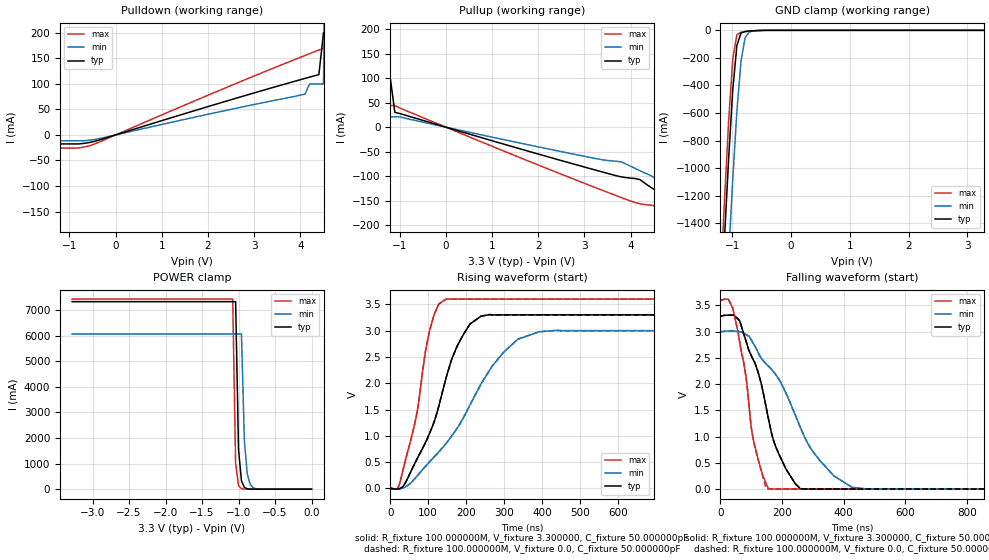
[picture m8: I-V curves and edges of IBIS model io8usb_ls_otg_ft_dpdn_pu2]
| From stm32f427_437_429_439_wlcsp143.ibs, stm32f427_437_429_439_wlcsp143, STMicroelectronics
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|   Model io8usb_ls_otg_ft_dpdn_pu2
[Model]  io8usb_ls_otg_ft_dpdn_pu2
Model_type I/O
Polarity   Non-Inverting
Enable   Active-Low
Vinl =   0.990000V
Vinh =   2.310000V
Vmeas =  1.650000V
Cref =   50.000000pF
Rref =   100.000000M
Vref =   0.0V
C_comp   8.255900pF   7.991100pF   8.650600pF
[Temperature Range]   25.000000   0.125000k   -40.000000
[Pullup Reference]   3.300000V   3.000000V   3.600000V
[Pulldown Reference]   0.0V   0.0V   0.0V
[POWER Clamp Reference]   3.300000V   3.000000V   3.600000V
[GND Clamp Reference]   0.0V   0.0V   0.0V
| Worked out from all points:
|   slope of the pulldown table from 0 to 0.495 V, typ, clamps not added: 35.6 ohm
|   slope of the pullup table from 0 to 0.495 V, typ, clamps not added: 36 ohm
|   GND clamp passes 1 mA (typ) near -0.52 V on its own axis
|   POWER clamp passes 1 mA (typ) near -0.81 V on its own axis
|   rising waveform, R_fixture 100.000000M, V_fixture 3.300000, C_fixture 50.000000pF: 20-80 % time 94.8ns typ, 161ns min, 53.8ns max; typ from 0 V to 3.3 V
|   rising waveform, R_fixture 100.000000M, V_fixture 0.0, C_fixture 50.000000pF: 20-80 % time 94.8ns typ, 162ns min, 53.7ns max; typ from 0 V to 3.3 V
|   falling waveform, R_fixture 100.000000M, V_fixture 3.300000, C_fixture 50.000000pF: 20-80 % time 97.5ns typ, 169ns min, 55.3ns max; typ from 3.3 V to 0 V
|   falling waveform, R_fixture 100.000000M, V_fixture 0.0, C_fixture 50.000000pF: 20-80 % time 97.5ns typ, 169ns min, 55.3ns max; typ from 3.3 V to 0 V
[Pulldown]
|Voltage   I(typ)   I(min)   I(max)
-3.3V     -181mA     -11.47mA   -25.86mA
-3.2V     -17.62mA   -11.47mA   -25.86mA
-600mV    -15.36mA   -10.76mA   -22.01mA
4.1V      110.7mA    80mA       155.6mA
4.2V      113.2mA    100mA      159.2mA
4.4V      118mA      100mA      166.2mA
4.5V      200mA      100mA      169.7mA
4.6V      200mA      1A         173.2mA
4.7V      200mA      1A         177mA
4.8V      1A         1A         200mA
5.4V      1A         1A         1A
6.6V      1A         1A         1A
[Pullup]
|Voltage   I(typ)   I(min)   I(max)
-3.3V     1A         1A         1A
-1.9V     1A         1A         1A
-1.8V     100mA      1A         1A
-1.7V     100mA      1A         100mA
-1.6V     100mA      1A         100mA
-1.5V     100mA      21mA       100mA
-1.3V     100mA      21mA       100mA
-1.2V     100mA      21mA       44mA
-1.1V     30mA       21mA       44mA
3.8V      -101.5mA   -71.06mA   -143.6mA
5V        -156.5mA   -125mA     -203mA
6.6V      -223mA     -162mA     -321mA
[GND_clamp]
|Voltage   I(typ)   I(min)   I(max)
-3.3V     -9.433A    -9.435A    -9.911A
-1.2V     -2.116A    -2.846A    -1.847A
-1.13V    -1.505A    -2.23A     -1.23A
-1.06V    -930.4mA   -1.637A    -658.9mA
-990mV    -432.7mA   -1.08A     -207.3mA
-920mV    -110.5mA   -590.3mA   -31.59mA
-850mV    -19.84mA   -226.8mA   -13.66mA
-780mV    -8.32mA    -54.05mA   -9.516mA
-710mV    -5.29mA    -11.97mA   -6.271mA
-640mV    -3.236mA   -4.296mA   -3.584mA
3.28V     0A         0A         0A
[POWER_clamp]
|Voltage   I(typ)   I(min)   I(max)
-3.28V    7.328A     6.064A     7.43A
-1.08V    7.328A     6.064A     7.43A
-1.04V    7.328A     6.064A     1.015A
-1V       1.545A     6.064A     138.6mA
-960mV    325.6mA    6.064A     18.93mA
-920mV    68.64mA    1.89A      2.585mA
-880mV    14.47mA    589mA      353uA
-840mV    3.05mA     183.6mA    105.9uA
-800mV    642.9uA    57.21mA    105.9uA
-720mV    28.59uA    5.557mA    105.9uA
0V        0A         0A         0A
[Ramp]
| variable   typ   min   max
dV/dt_r  1.45447/0.11070u   1.20651/0.19758u   1.71898/64.82544n
dV/dt_f  1.45908/95.28125n   1.20980/0.16655u   1.72159/55.34417n
R_load = 100.000000
[Rising Waveform]
R_fixture= 100.000000M
V_fixture= 3.300000
V_fixture_min= 3.000000
V_fixture_max= 3.600000
C_fixture= 50.000000pF
|time   V(typ)   V(min)   V(max)
0s        106.1uV    63.26uV    178.2uV
25.36ns   -431.7uV   -4.181mV   112.8mV
69.4ns    545.2mV    227.1mV    1.402V
104.1ns   1.058V     510.2mV    3.014V
146.8ns   2.094V     854.7mV    3.597V
192.2ns   2.92V      1.337V     3.599V
238.9ns   3.273V     1.983V     3.6V
336.3ns   3.3V       2.838V     3.6V
392.4ns   3.3V       2.978V     3.6V
1.333us   3.3V       3V         3.6V
[Rising Waveform]
R_fixture= 100.000000M
V_fixture= 0.0
V_fixture_min= 0.0
V_fixture_max= 0.0
C_fixture= 50.000000pF
|time   V(typ)   V(min)   V(max)
0s        104.9uV    61.81uV    177.3uV
25.36ns   -442.7uV   -4.191mV   112.8mV
69.4ns    545.2mV    227.1mV    1.404V
104.1ns   1.058V     510.1mV    3.011V
146.8ns   2.094V     854.7mV    3.597V
192.2ns   2.92V      1.337V     3.6V
238.9ns   3.273V     1.983V     3.6V
335ns     3.3V       2.83V      3.6V
392.4ns   3.3V       2.978V     3.6V
1.333us   3.3V       3V         3.6V
[Falling Waveform]
R_fixture= 100.000000M
V_fixture= 3.300000
V_fixture_min= 3.000000
V_fixture_max= 3.600000
C_fixture= 50.000000pF
|time   V(typ)   V(min)   V(max)
0s        3.3V       3V         3.6V
40.04ns   3.313V     3.012V     3.447V
82.75ns   2.825V     2.945V     2.15V
105.4ns   2.476V     2.788V     979.9mV
156.2ns   1.33V      2.338V     11.44mV
190.9ns   651.2mV    2.081V     -468.2uV
258.9ns   7.023mV    1.181V     193.7uV
325.7ns   165.3uV    522.8mV    190.8uV
427.1ns   107.7uV    31.8mV     176.9uV
1.333us   106.2uV    24.43uV    167uV
[Falling Waveform]
R_fixture= 100.000000M
V_fixture= 0.0
V_fixture_min= 0.0
V_fixture_max= 0.0
C_fixture= 50.000000pF
|time   V(typ)   V(min)   V(max)
0s        3.3V       3V         3.6V
41.37ns   3.313V     3.012V     3.416V
82.75ns   2.825V     2.945V     2.15V
105.4ns   2.476V     2.788V     980.3mV
152.2ns   1.446V     2.362V     8.278mV
190.9ns   651.2mV    2.081V     344.1uV
258.9ns   7.204mV    1.181V     184.8uV
324.3ns   166.7uV    532.2mV    176.8uV
427.1ns   106.5uV    33.12mV    178.2uV
1.333us   105uV      22.53uV    176.5uV
